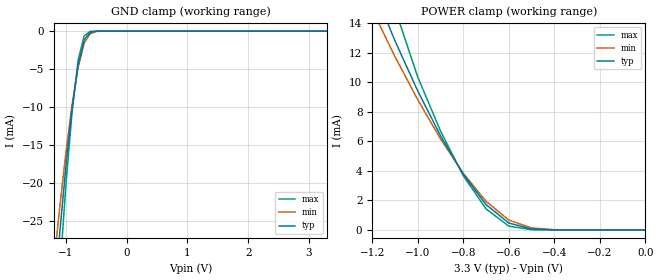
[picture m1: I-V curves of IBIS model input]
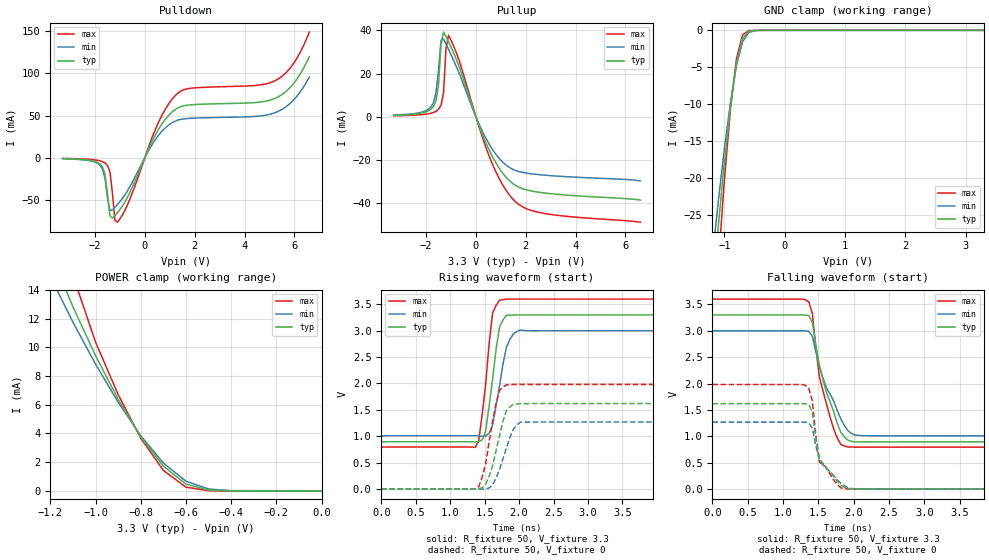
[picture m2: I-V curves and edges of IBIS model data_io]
[IBIS Ver]   3.2
[Comment Char]   |_char
[File name]   as7c34098a_tsopi.ibs
[File Rev]   1.1
[Date]   July 29, 2004 10:20:13 AM
[Source]
Alliance Semiconductor Corporation
[Notes]
This model  is for TSOP package & Industrial operation.
[Disclaimer]
Data is for modelling purpose only & not guranteed.
[Copyright]
Alliance Semiconductor Corporation
| TSOP Package.
[Component]   7c34098a_tsopi
Si_location Pin
Timing_location Pin
[Manufacturer]   Alliance Semiconductor Corporation
[Package]
R_pkg   320m   170.7m   426.1m
L_pkg   4.9nH   3.2nH   6.505nH
C_pkg   0.9pF   0.51pF   1.215pF
[Pin] signal_name   model_name
1   A0   input
2   A1   input
3   A2   input
4   A3   input
5   A4   input
6   NCE   input
7   IO1   data_io
8   IO2   data_io
9   IO3   data_io
10   IO4   data_io
11   VCC   POWER
12   GND   GND
13   IO5   data_io
14   IO6   data_io
15   IO7   data_io
16   IO8   data_io
17   NWE   input
18   A5   input
19   A6   input
20   A7   input
21   A8   input
22   A9   input
23   A10   input
24   A11   input
25   A12   input
26   A13   input
27   A14   input
28   NC   NC
29   IO9   data_io
30   IO10   data_io
31   IO11   data_io
32   IO12   data_io
33   VCC   POWER
34   GND   GND
35   IO13   data_io
36   IO14   data_io
37   IO15   data_io
38   IO16   data_io
39   NLB   input
40   NUB   input
41   NOE   input
42   A15   input
43   A16   input
44   A17   input
| Models and submodels in the file (2): input (Input), data_io (I/O)
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[Model]   input
Model_type Input
Vinh=2V
Vinl=0.8V
C_comp   4.5pF   4.5pF   4.5pF
[Temperature Range] 25   85   -40
[Voltage Range]   3.3   3.0   3.6
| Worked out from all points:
|   GND clamp passes 1 mA (typ) near -0.69 V on its own axis
|   POWER clamp passes 1 mA (typ) near -0.64 V on its own axis
[GND Clamp]
-3.3V     -5.963A    -5.758A    -6.71A
-1.2V     -35.86mA   -30.72mA   -72.08mA
-1.1V     -26.38mA   -23.03mA   -31.63mA
-1V       -17.75mA   -15.98mA   -20.16mA
-900mV    -10.25mA   -9.754mA   -10.71mA
-800mV    -4.452mA   -4.757mA   -3.831mA
-700mV    -1.141mA   -1.578mA   -626.8uA
-600mV    -151uA     -315.5uA   -43.02uA
-500mV    -13.23uA   -43.92uA   -1.67uA
-400mV    -845.7nA   -4.852uA   -42.98nA
3.3V      69.07pA    1.836uA    59.97pA
[POWER Clamp]
-3.3V     5.963A     5.758A     6.709A
-1.2V     16.57mA    14.94mA    55.98mA
-1.1V     12.83mA    11.76mA    15.01mA
-1V       9.429mA    8.836mA    10.37mA
-900mV    6.388mA    6.181mA    6.715mA
-800mV    3.775mA    3.845mA    3.679mA
-700mV    1.722mA    1.942mA    1.431mA
-600mV    472uA      674.7uA    260.2uA
-500mV    61.49uA    135.7uA    16.56uA
-400mV    5.003uA    17.74uA    603.1nA
0V        69.07pA    221.7pA    72.01pA
[Model]   data_io
Model_type I/O
Enable Active-High
Polarity Non-Inverting
Vinh=2V
Vinl=0.8V
Vref=1.728V
Vmeas=1.5V
Rref=168
Cref=5pF
C_comp   4.5pF   4.5pF   4.5pF
[Temperature Range] 25   85   -40
[Voltage Range]   3.3   3.0   3.6
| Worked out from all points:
|   slope of the pulldown table from 0 to 0.495 V, typ, clamps not added: 16 ohm
|   slope of the pullup table from 0 to 0.495 V, typ, clamps not added: 34.3 ohm
|   GND clamp passes 1 mA (typ) near -0.69 V on its own axis
|   POWER clamp passes 1 mA (typ) near -0.64 V on its own axis
|   falling waveform, R_fixture 50, V_fixture 3.3: 20-80 % time 283ps typ, 329ps min, 230ps max; typ from 3.3 V to 0.895 V
|   falling waveform, R_fixture 50, V_fixture 0: 20-80 % time 236ps typ, 285ps min, 197ps max; typ from 1.62 V to 0.001 V
|   rising waveform, R_fixture 50, V_fixture 3.3: 20-80 % time 142ps typ, 160ps min, 131ps max; typ from 0.894 V to 3.3 V
|   rising waveform, R_fixture 50, V_fixture 0: 20-80 % time 184ps typ, 200ps min, 162ps max; typ from 0 V to 1.62 V
[Pullup]
-3.3V     659uA      791uA      435uA
-1.8V     3.486mA    4.587mA    1.615mA
-1.6V     7.4mA      11.28mA    2.502mA
-1.5V     14.72mA    21.58mA    3.42mA
-1.4V     33.46mA    35.44mA    5.292mA
-1.3V     39.19mA    35.97mA    10.92mA
-1.2V     37.2mA     33.69mA    31.42mA
-1.1V     34.82mA    31.25mA    37.72mA
500mV     -14.56mA   -12.01mA   -17.24mA
1.6V      -31.87mA   -24.92mA   -39.46mA
2.8V      -35.38mA   -27.11mA   -44.89mA
6.6V      -38.58mA   -29.67mA   -48.84mA
[Pulldown]
-3.3V     -1.242mA   -1.364mA   -938uA
-1.8V     -7.54mA    -9.121mA   -3.789mA
-1.6V     -19.38mA   -24.68mA   -6.262mA
-1.5V     -42.76mA   -48.09mA   -9.289mA
-1.4V     -69.26mA   -62.73mA   -16.7mA
-1.2V     -68.87mA   -59.04mA   -74.61mA
-1.1V     -65.45mA   -55.76mA   -76.68mA
400mV     25.83mA    20.49mA    32.03mA
1.2V      56.73mA    43.15mA    73.07mA
5.2V      70.16mA    53.14mA    91.06mA
5.9V      85.65mA    66.43mA    109.1mA
6.6V      120mA      95.68mA    149.1mA
[GND Clamp]
-3.3V     -5.963A    -5.758A    -6.71A
-1.2V     -35.86mA   -30.72mA   -72.08mA
-1.1V     -26.38mA   -23.03mA   -31.63mA
-1V       -17.75mA   -15.98mA   -20.16mA
-900mV    -10.25mA   -9.754mA   -10.71mA
-800mV    -4.452mA   -4.757mA   -3.831mA
-700mV    -1.141mA   -1.578mA   -626.8uA
-600mV    -151uA     -315.5uA   -43.02uA
-500mV    -13.23uA   -43.92uA   -1.67uA
-400mV    -845.7nA   -4.852uA   -42.98nA
3.3V      69.07pA    1.836uA    59.97pA
[POWER Clamp]
-3.3V     5.963A     5.758A     6.709A
-1.2V     16.57mA    14.94mA    55.98mA
-1.1V     12.83mA    11.76mA    15.01mA
-1V       9.429mA    8.836mA    10.37mA
-900mV    6.388mA    6.181mA    6.715mA
-800mV    3.775mA    3.845mA    3.679mA
-700mV    1.722mA    1.942mA    1.431mA
-600mV    472uA      674.7uA    260.2uA
-500mV    61.49uA    135.7uA    16.56uA
-400mV    5.003uA    17.74uA    603.1nA
0V        69.07pA    221.7pA    72.01pA
[Falling Waveform]
R_fixture=50
V_fixture=3.3
V_fixture_min=3.0
V_fixture_max=3.6
0s        3.3V       3V         3.6V
1.364ns   3.289V     2.988V     3.547V
1.414ns   3.16V      2.897V     3.33V
1.515ns   2.334V     2.317V     2.116V
1.616ns   1.823V     1.91V      1.601V
1.717ns   1.46V      1.663V     1.136V
1.818ns   1.072V     1.326V     845.3mV
1.869ns   986.9mV    1.2V       816.1mV
2.121ns   895.4mV    1.014V     795mV
5ns       895.3mV    1.009V     794.8mV
[Falling Waveform]
R_fixture=50
V_fixture=0
V_fixture_min=0
V_fixture_max=0
0s        1.619V     1.269V     1.982V
1.313ns   1.617V     1.267V     1.967V
1.364ns   1.606V     1.256V     1.909V
1.414ns   1.457V     1.151V     1.676V
1.465ns   949.4mV    809.2mV    997.3mV
1.515ns   569.1mV    543.8mV    509.4mV
1.616ns   403mV      381.2mV    400.8mV
1.818ns   70.45mV    105.2mV    23.83mV
2.02ns    -1.233mV   1.801mV    918.7uV
5ns       903uV      773.7uV    654.7uV
[Rising Waveform]
R_fixture=50
V_fixture=3.3
V_fixture_min=3.0
V_fixture_max=3.6
0s        894mV      1.008V     794.1mV
1.364ns   890.5mV    1.01V      786.8mV
1.414ns   897.3mV    1.008V     920.4mV
1.515ns   1.101V     1.005V     1.995V
1.566ns   1.582V     1.058V     2.769V
1.616ns   2.091V     1.213V     3.34V
1.717ns   3.076V     1.968V     3.576V
1.818ns   3.293V     2.696V     3.597V
2.02ns    3.299V     3.01V      3.599V
5ns       3.299V     2.999V     3.599V
[Rising Waveform]
R_fixture=50
V_fixture=0
V_fixture_min=0
V_fixture_max=0
0s        0V         0V         0V
1.414ns   4.37mV     548.3uV    45.05mV
1.515ns   89.09mV    815.1uV    481.6mV
1.566ns   246mV      20.6mV     899.1mV
1.667ns   735.6mV    212.5mV    1.628V
1.717ns   1.019V     372.7mV    1.871V
1.818ns   1.489V     785.4mV    1.973V
1.919ns   1.605V     1.135V     1.98V
2.02ns    1.616V     1.266V     1.981V
5ns       1.619V     1.269V     1.982V
[Ramp]
R_load=50
dV/dt_r   9.712E-1/1.779E-10   7.613E-1/1.950E-10   1.189E+0/1.554E-10
dV/dt_f   1.443E+0/2.832E-10   1.194E+0/3.263E-10   1.683E+0/2.305E-10
|[End   data_io
